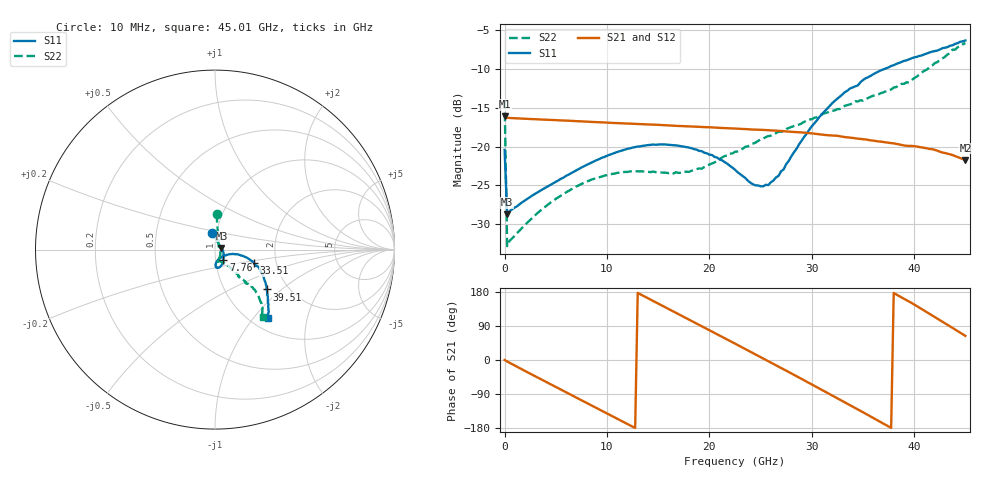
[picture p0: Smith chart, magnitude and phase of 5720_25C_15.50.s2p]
! Device:  ADRF5720
! Description: 0.5dB LSB GaAs MMIC 6-bit Digital Attenuator
! Frequency:  0.000009 -  40 GHz
! Ports:
!	RF1	= Port 1
!	RF2	= Port 2
! Vdd:  3.3 Volt
! Vss:  -3.3 Volt
! Control:  0/3.3 Volt
! State:  15.50 dB attenuation
! Data:  The device was measured using G-S-G Probes on a matrix board.
!  Data was collected using an calibrated 4 port network analyzer.
!  The reference plane for this measurement is at the launchers.
! Note:  Analog Devices supplies this data as a sample of measured data
!  for this product.  Your particular data for this product may vary.
!  Data was taken at 25 degrees C.
!  Analog Devices reserves the right to change this data at anytime.
# GHZ S DB R 45.0
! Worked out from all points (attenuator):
!   181 points, 10 MHz to 45.01 GHz, reference 45 ohm
!   highest |S21| = -16.12 dB at 10 MHz (marker M1); lowest = -21.7 dB at 45.01 GHz (marker M2)
!   lowest |S11| = -28.7 dB at 260 MHz (marker M3), VSWR 1.08, Z = 48.3 + j0.808 ohm
!   |S11| at or under -10 dB: start of sweep to 37.14 GHz
!   |S22| runs from -32.8 to -6.7 dB; largest |S21 - S12| = 0.0002
!   S11 on the Smith chart (normalised r, x): 10 MHz: 0.95, +0.18; 7.76 GHz: 1.09, -0.13; 33.51 GHz: 1.53, -0.24; 39.51 GHz: 1.56, -0.80; 45.01 GHz: 1.19, -1.18
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0.01  -20.43 100.4  -16.12 0.0  -16.12 0.0  -14.03 87.5
0.26  -28.73 13.2  -16.31 -3.9  -16.31 -3.9  -32.81 20.3
1.26  -27.64 -2.8  -16.38 -18.4  -16.38 -18.4  -31.06 -7.6
4.26  -25.08 -30.3  -16.56 -60.7  -16.56 -60.7  -27.45 -46.7
7.76  -22.53 -51.4  -16.78 -109.6  -16.78 -109.6  -24.65 -68.8
11.76  -20.40 -68.8  -17.03 -165.5  -17.03 -165.4  -23.27 -80.2
15.26  -19.72 -80.3  -17.23 145.4  -17.23 145.4  -23.33 -80.1
18.01  -20.13 -86.5  -17.41 106.8  -17.42 106.9  -23.26 -70.4
19.01  -20.56 -87.5  -17.47 92.7  -17.47 92.7  -22.82 -65.6
21.26  -21.78 -87.1  -17.61 60.9  -17.61 60.9  -21.40 -58.2
22.76  -23.29 -82.7  -17.71 39.7  -17.71 39.8  -20.62 -54.3
24.51  -24.99 -63.7  -17.82 15.0  -17.82 15.0  -19.50 -52.0
25.76  -24.95 -44.7  -17.90 -3.0  -17.91 -2.9  -18.66 -51.1
27.26  -22.94 -23.8  -18.02 -24.6  -18.03 -24.6  -18.00 -49.2
30.26  -17.00 -12.0  -18.35 -68.2  -18.35 -68.1  -16.30 -48.7
32.01  -14.42 -14.8  -18.59 -93.5  -18.59 -93.5  -15.42 -48.7
33.51  -12.80 -19.4  -18.82 -115.8  -18.82 -115.8  -14.66 -48.1
35.51  -11.09 -25.1  -19.14 -145.6  -19.14 -145.5  -13.75 -48.0
37.76  -9.64 -32.4  -19.56 -179.2  -19.56 -179.1  -12.66 -46.6
39.51  -8.78 -37.5  -19.92 154.3  -19.93 154.4  -11.76 -47.0
42.26  -7.66 -44.6  -20.53 109.2  -20.53 109.3  -9.15 -46.5
45.01  -6.36 -52.5  -21.74 63.7  -21.74 63.7  -6.69 -54.4
